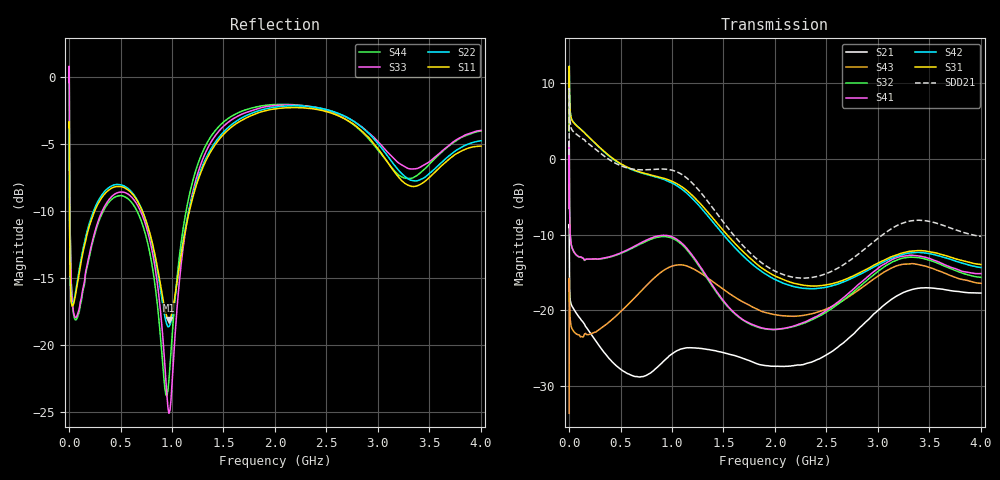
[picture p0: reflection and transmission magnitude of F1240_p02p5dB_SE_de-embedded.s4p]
! Integrated Device Technology
! Corporate Headquarters
! 6024 Silver Creek Valley Road
! San Jose, CA 95138  USA
! Phone:  1-408-284-8200
! Toll Free:  1-800-223-1366
! Webpage:  http://www.idt.com/
! Timing and RF Division
! 515 Groton Road, Suite 102
! Westford, MA 01886-6024
! Device:  F1240
! Description: Dual Intermediate Frequency Digital Variable Gain Amplifier
! Frequency:  10.0 -  500.00 MHz
! Package:  5x5 mm QFN Plastic Package: 32 pin
! Ports:  8 RF, 20 DC
!  Pin  1  = GA3 / Data  Pin 17  = RF OUT_B+
!  Pin  2  = GA4 / CLK  Pin 18  = RF OUT_B-
!  Pin  3  = GA5  Pin 19  = STBY_B
!  Pin  4  = VMODE  Pin 20  = Ground
!  Pin  5  = No Connect  Pin 21  = Ground
!  Pin  6  = GB5  Pin 22  = STB_A
!  Pin  7  = GB4  Pin 23  = RF OUT_A-  = Port 4
!  Pin  8  = GB3  Pin 24  = RF OUT_A+  = Port 3
!  Pin  9  = GB2  Pin 25  = GA0
!  Pin 10  = GB1  Pin 26  = ISET_A
!  Pin 11  = RF IN_B+  Pin 27  = VCC
!  Pin 12  = RF IN_B-  Pin 28  = Ground
!  Pin 13  = Ground  Pin 29  = RF IN_A-  = Port 2
!  Pin 14  = VCC  Pin 30  = RF IN_A+  = Port 1
!  Pin 15  = ISET_B  Pin 31  = GA1
!  Pin 16  = GB0  Pin 32  = GA2 / CSb
! Gain  = +19.5 dB
! State  = 1
! Voltage  = +5.00 V
! Current  = 85.292 mA (one channel only)
! Temperture  =  +25 C
! Test Date  =  2017-10-18
! Board  =  EB4031
! Data:  The device was measured on a custom evaluation board which has
!  individual transmission lines to the RF pins.  Data was collected
!  using a calibrated network analyzer.  The evaluation board was
!  de-embedded using Automatic Fixture Removal.
!  The reference plane is the edge of the package pin.
!  Only Channel A was measured.
!  This data is in single-ended operation.  If your needs are balanced
!  or differential S-parameters then this file needs to be used a
!  linear simulator.
! File Date:  2017-11-10  MJV
! Note:
!  Integrated Device Technology supplies this data as a sample of measured
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# Hz S dB R 100
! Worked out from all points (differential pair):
!   410 points, 500 kHz to 4 GHz, reference 100 ohm
!   strongest paths, dB at 500 kHz, 930 MHz, 1.96 GHz, 2.98 GHz, 4 GHz:
!     S31: 3.7, -2.6, -15.2, -13.9, -13.9
!     S42: 3.7, -2.8, -15.6, -14.1, -14.3
!     S41: -6.5, -10.1, -22.5, -14.7, -15.1
!     S32: -6.5, -10.3, -22.5, -15.1, -15.6
!     S43: -33.6, -14.6, -20.5, -15.7, -16.4
!     S21: -9.1, -26.6, -27.4, -20.3, -17.7
!   taken as a pair (ports 1,2 in; 3,4 out), SDD21 dB: 0.5, -1.4, -14.5, -10.7, -10.2
!   lowest |S11| = -18.1 dB at 970 MHz (marker M1), VSWR 1.28, Z = 79.4 - j8.48 ohm
!   |S11| at or under -10 dB: 4.396 MHz to 248.9 MHz (244.5 MHz wide, 193 % of centre); 711.9 MHz to 1.169 GHz (456.9 MHz wide, 48.6 % of centre)
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500000  -3.76 -5.5  -9.05 -5.7  -29.23 81.8  -39.35 79.4
        -9.06 -5.7  -3.76 -5.5  -39.35 78.4  -29.23 82.9
        3.72 -106.3  -6.52 -107.5  -0.38 1.1  -33.57 -54.0
        -6.54 -106.4  3.70 -105.1  -33.58 -54.2  -0.39 3.4
2500000  -5.90 -47.8  -12.57 -45.9  -18.52 27.7  -30.52 3.0
         -12.58 -45.9  -5.87 -47.8  -30.47 2.7  -18.52 28.0
         11.64 -179.9  0.29 157.6  -0.87 -55.3  -15.78 -153.6
         0.24 157.8  11.63 -179.6  -15.76 -153.7  -0.92 -55.0
4500000  -10.18 -56.2  -16.63 -37.5  -18.53 11.5  -33.02 -11.0
         -16.64 -37.6  -10.14 -56.4  -32.99 -11.2  -18.54 11.5
         8.98 163.2  -5.40 139.3  -5.04 -81.0  -18.27 175.2
         -5.44 139.4  8.98 163.4  -18.24 175.2  -5.10 -81.0
1.8e8  -11.59 -115.8  -22.46 -54.4  -20.66 -46.6  -35.90 -20.1
       -22.48 -54.3  -11.37 -117.1  -35.96 -19.5  -20.68 -46.8
       3.03 113.7  -13.24 68.0  -13.85 -135.2  -23.28 101.7
       -13.22 67.9  3.03 112.9  -23.21 101.2  -14.01 -134.8
5.3e8  -8.23 -166.9  -28.10 -99.1  -22.10 -111.4  -32.52 -72.1
       -28.05 -98.1  -8.10 -168.5  -32.69 -70.1  -22.27 -111.9
       -0.86 22.5  -12.33 -55.6  -8.59 -171.4  -20.04 7.1
       -12.24 -56.9  -0.91 21.3  -19.81 6.8  -8.89 -171.7
9.7e8  -18.13 -154.9  -26.30 -131.1  -21.12 152.9  -29.86 -160.3
       -26.03 -134.1  -18.64 -153.1  -29.92 -154.4  -21.63 151.6
       -2.80 -86.9  -10.34 168.6  -25.11 -153.6  -14.62 -106.3
       -10.16 165.1  -2.99 -89.4  -14.32 -106.7  -22.62 -123.5
4e9  -5.14 -140.7  -17.75 103.3  -24.11 -47.4  -25.01 -30.5
     -17.71 103.1  -4.74 -139.1  -25.88 -15.0  -25.86 -40.9
     -13.95 34.6  -15.64 -70.5  -3.97 -134.9  -17.74 67.5
     -15.14 -84.2  -14.34 40.5  -16.43 57.9  -4.01 -144.4
